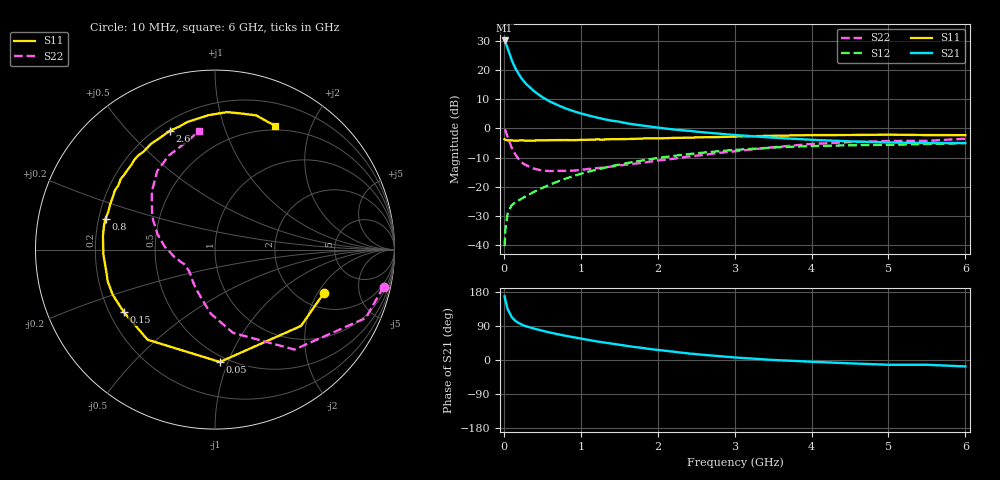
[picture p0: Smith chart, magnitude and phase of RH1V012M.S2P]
! SIEMENS Small Signal Semiconductors
! BFR106
! Si NPN RF Bipolar Junction Transistor in SOT23
! VCE = 1 V  IC = 12 mA
! Common Emitter S-Parameters:  August  1996
# GHz  S  MA  R  50
!  f  S11  S21  S12  S22
! GHz  MAG  ANG  MAG  ANG  MAG  ANG  MAG  ANG
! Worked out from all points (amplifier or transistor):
!   36 points, 10 MHz to 6 GHz, reference 50 ohm
!   highest |S21| = 30.1 dB at 10 MHz (marker M1)
!   |S21| within 3 dB of that: start of sweep to 53.18 MHz
!   unconditionally stable (mu >= 1): 419.9 MHz to 2.998 GHz; 4.049 GHz to end of sweep
!   at 250 MHz: K = 0.78, MSG = 20.1 dB, |S12| = -23.7 dB
!   at 1.4 GHz: K = 1.11, MAG = 5.8 dB, |S12| = -12.9 dB
!   at 6 GHz: K = 1.03, MAG = -1.0 dB, |S12| = -5.0 dB
!   S11 on the Smith chart (normalised r, x): 10 MHz: 2.72, -2.27; 50 MHz: 0.45, -0.94; 150 MHz: 0.26, -0.29; 800 MHz: 0.23, +0.13; 2.6 GHz: 0.25, +0.66; 6 GHz: 0.45, +1.51
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0.01  0.6539 -21.5  31.99 167.9  0.0097 81.9  0.9616 -12.4
0.02  0.6407 -41.6  30.35 157.9  0.0185 72.1  0.9226 -24.4
0.05  0.6266 -87.5  23.28 133.9  0.0359 54.2  0.7116 -51.5
0.1  0.627 -126.8  15.06 113.7  0.0482 43.7  0.4744 -77.8
0.15  0.6161 -145.8  10.66 103.1  0.0547 41.9  0.3575 -93.8
0.2  0.623 -156.2  8.252 96.8  0.0596 43.6  0.291 -103.7
0.25  0.6235 -163.4  6.645 91.8  0.0652 45.0  0.2518 -112.9
0.3  0.6178 -168.6  5.594 88.4  0.071 47.5  0.2316 -119.4
0.4  0.6219 -176.9  4.259 82.5  0.0834 51.1  0.204 -130.1
0.5  0.6243 177.4  3.43 77.3  0.096 53.8  0.1903 -137.5
0.6  0.6294 172.5  2.886 72.5  0.1098 55.5  0.1867 -142.6
0.7  0.6325 167.7  2.505 68.0  0.1236 56.4  0.1881 -147.2
0.8  0.6338 164.2  2.21 64.0  0.1381 56.9  0.1888 -151.6
1.1  0.6407 152.6  1.668 52.9  0.1822 56.2  0.2029 -160.2
1.3  0.6464 146.4  1.445 46.2  0.2116 54.6  0.2145 -165.9
1.6  0.6596 137.3  1.224 37.2  0.2554 51.4  0.2413 -173.5
2.2  0.6886 121.1  0.962 22.0  0.3387 43.0  0.3029 170.8
2.6  0.7082 110.8  0.856 13.5  0.3871 36.6  0.3526 159.9
3.5  0.7498 92.8  0.697 0.1  0.472 22.0  0.4773 137.6
4.5  0.7727 78.6  0.601 -8.8  0.5155 7.1  0.5835 116.3
5.5  0.7703 67.7  0.563 -12.6  0.5428 -2.0  0.6152 105.7
6  0.7676 64.0  0.564 -17.0  0.5597 -8.6  0.6672 97.7
